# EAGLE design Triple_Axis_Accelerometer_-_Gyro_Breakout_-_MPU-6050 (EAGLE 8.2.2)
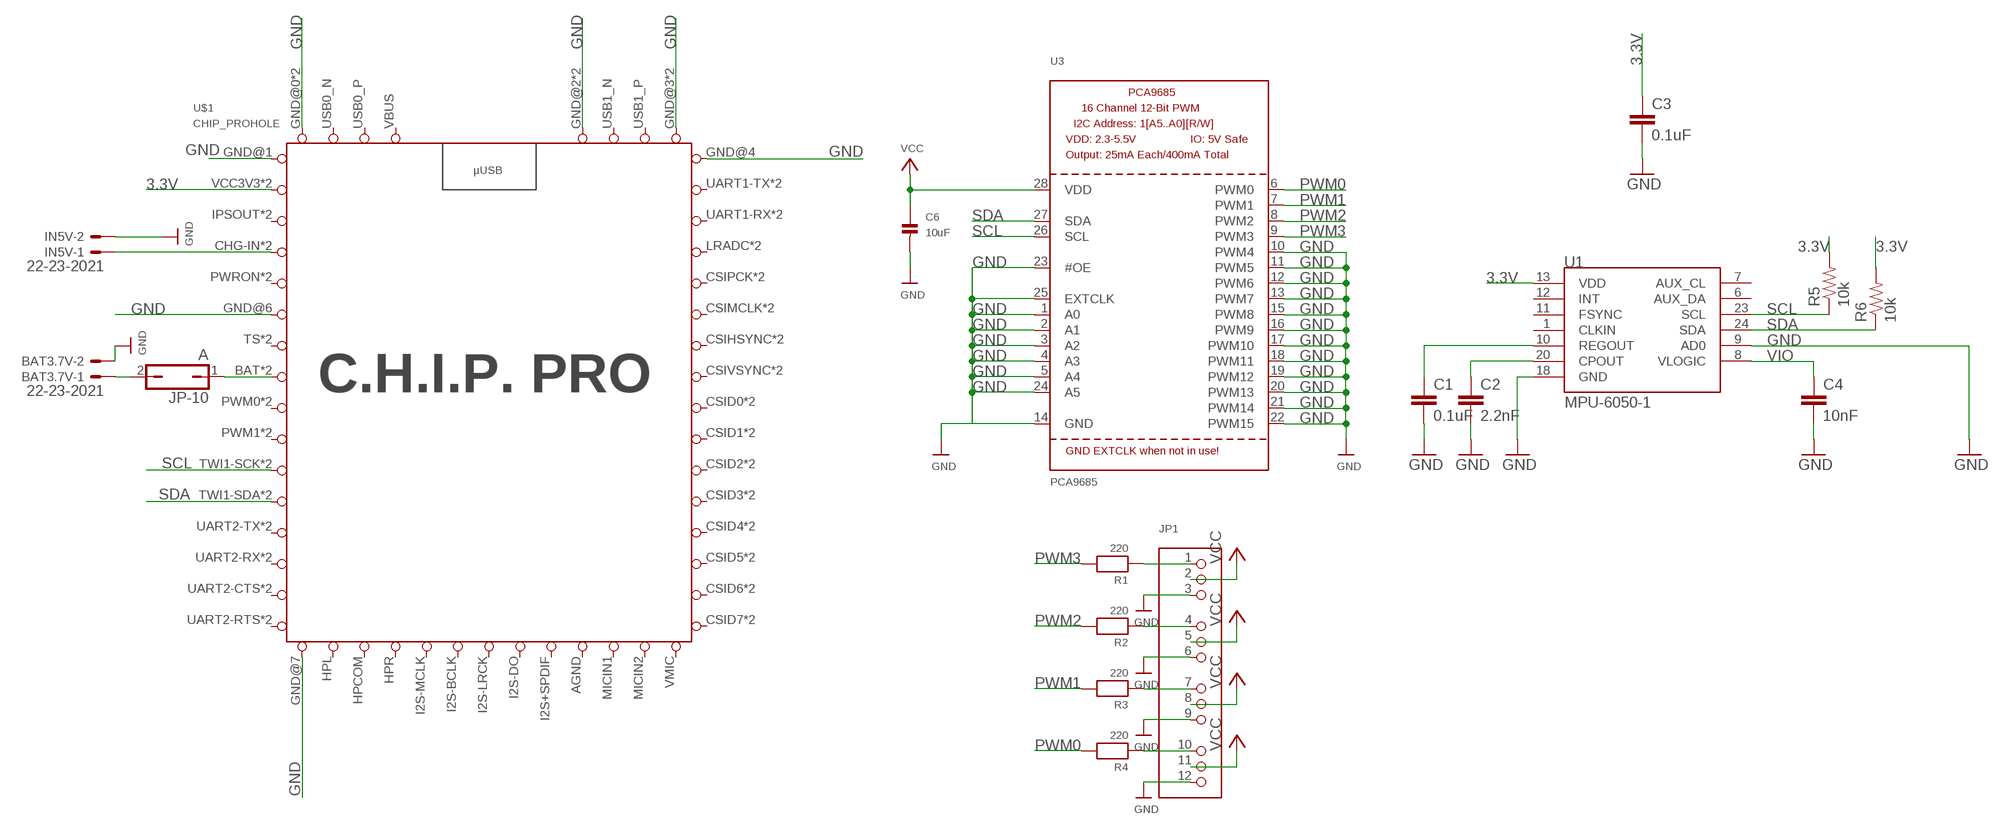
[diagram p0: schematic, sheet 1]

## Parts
BAT3.7V  22-23-2021  [22-23-2021]
C1  0.1uF  CAP0603-CAP  [0603-CAP]
C2  2.2nF  CAP0603-CAP  [0603-CAP]
C3  0.1uF  CAP0603-CAP  [0603-CAP]
C4  10nF  CAP0603-CAP  [0603-CAP]
C6  10uF  CAP_CERAMIC0805  [0805]
IN5V  22-23-2021  [22-23-2021]
JP1  HEADER-3X04  [3X04]
JP-10  A  JP1Q  [JP1]
R1  220  RESISTOR0805  [0805]
R2  220  RESISTOR0805  [0805]
R3  220  RESISTOR0805  [0805]
R4  220  RESISTOR0805  [0805]
R5  10k  R-US_R0805  [R0805]
R6  10k  R-US_R0805  [R0805]
U1  MPU-6050-1  [QFN-24-4MM2]
U3  PCA9685  [TSSOP28]
U$1  CHIP_PROHOLE  [CHIP_PRO_HOLE]

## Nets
3.3V: C3.1 R5.2 R6.2 U1.13(VDD) U$1.VCC3V3 U$1.VCC3V3-1(VCC3V3)
GND: BAT3.7V.2 C1.2 C2.2 C3.2 C4.2 C6.2 IN5V.2 JP1.3 JP1.6 JP1.9 JP1.12 U1.9(AD0) U1.18(GND) U3.1(A0) U3.2(A1) U3.3(A2) U3.4(A3) U3.5(A4) U3.10(PWM4) U3.11(PWM5) U3.12(PWM6) U3.13(PWM7) U3.14(GND) U3.15(PWM8) U3.16(PWM9) U3.17(PWM10) U3.18(PWM11) U3.19(PWM12) U3.20(PWM13) U3.21(PWM14) U3.22(PWM15) U3.23(#OE) U3.24(A5) U3.25(EXTCLK) U$1.GND@0(GND) U$1.GND@0-1(GND) U$1.GND@1(GND) U$1.GND@2(GND) U$1.GND@2-1(GND) U$1.GND@3(GND) U$1.GND@3-1(GND) U$1.GND@4(GND) U$1.GND@6(GND) U$1.GND@7(GND)
N$1: JP1.1 R1.1
N$2: JP1.4 R2.1
N$3: C2.1 U1.20(CPOUT)
N$4: JP1.7 R3.1
N$5: C1.1 U1.10(REGOUT)
N$6: JP1.10 R4.1
N$9: IN5V.1 U$1.CHG-IN U$1.CHG-IN-1(CHG-IN)
PWM0: R4.2 U3.6(PWM0)
PWM1: R3.2 U3.7(PWM1)
PWM2: R2.2 U3.8(PWM2)
PWM3: R1.2 U3.9(PWM3)
SCL: R5.1 U1.23(SCL) U3.26(SCL) U$1.TWI1-SCK U$1.TWI1-SCK-1(TWI1-SCK)
SDA: R6.1 U1.24(SDA) U3.27(SDA) U$1.TWI1-SDA U$1.TWI1-SDA-1(TWI1-SDA)
VCC: BAT3.7V.1 C6.1 JP1.2 JP1.5 JP1.8 JP1.11 JP-10.1 JP-10.2 U3.28(VDD) U$1.BAT U$1.BAT-1(BAT)
VIO: C4.1 U1.8(VLOGIC)
Unconnected: U1.1(CLKIN) U1.6(AUX_DA) U1.7(AUX_CL) U1.11(FSYNC) U1.12(INT) U$1.CSID0 U$1.CSID0-1(CSID0) U$1.CSID1 U$1.CSID1-1(CSID1) U$1.CSID2 U$1.CSID2-1(CSID2) U$1.CSID3 U$1.CSID3-1(CSID3) U$1.CSID4 U$1.CSID4-1(CSID4) U$1.CSID5 U$1.CSID5-1(CSID5) U$1.CSID6 U$1.CSID6-1(CSID6) U$1.CSID7 U$1.CSID7-1(CSID7) U$1.CSIHSYNC U$1.CSIHSYNC-1(CSIHSYNC) U$1.CSIMCLK U$1.CSIMCLK-1(CSIMCLK) U$1.CSIPCK U$1.CSIPCK-1(CSIPCK) U$1.CSIVSYNC U$1.CSIVSYNC-1(CSIVSYNC) U$1.HPCOM U$1.HPL U$1.HPR U$1.I2S+SPDIF(I2SSPDIF) U$1.I2S-BCLK(I2SBCLK) U$1.I2S-DO(I2SDO) U$1.I2S-LRCK(I2SLRCK) U$1.I2S-MCLK(I2SMCLK) U$1.LRADC U$1.LRADC-1(LRADC) U$1.MICIN1 U$1.MICIN2 U$1.PWM0 U$1.PWM0-1(PWM0) U$1.PWM1 U$1.PWM1-1(PWM1) U$1.PWRON U$1.PWRON-1(PWRON) U$1.TS U$1.TS-1(TS) U$1.UART1-RX U$1.UART1-RX-1(UART1-RX) U$1.UART1-TX U$1.UART1-TX-1(UART1-TX) U$1.UART2-CTS U$1.UART2-CTS-1(UART2-CTS) U$1.UART2-RTS U$1.UART2-RTS-1(UART2-RTS) U$1.UART2-RX U$1.UART2-RX-1(UART2-RX) U$1.UART2-TX U$1.UART2-TX-1(UART2-TX) U$1.USB0_N U$1.USB0_P U$1.USB1_N U$1.USB1_P U$1.VMIC

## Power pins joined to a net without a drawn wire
AGND: U$1.AGND
IPSOUT: U$1.IPSOUT U$1.IPSOUT-1(IPSOUT)
VBUS: U$1.VBUS

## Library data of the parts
BAT3.7V IN5V = con-molex:22-23-2021: .100" (2.54mm) Center Header - 2 Pin; MF: MOLEX; MPN: 22-23-2021; OC_FARNELL: 1462926; OC_NEWARK: 25C3832
C1-C4 = SparkFun:CAP: Capacitor
C6 = microbuilder:CAP_CERAMIC: Ceramic Capacitors
JP1 = microbuilder:HEADER-3X04
JP-10 = jumper:JP1Q: JUMPER
R1-R4 = microbuilder:RESISTOR: Resistors
R5 R6 = rcl:R-US_: RESISTOR, American symbol
U1 = Testing:MPU-6050
U3 = microbuilder:PCA9685: PCA9685 - 16 Channel 12-Bit I2C PWM Controller 5.0V tolerant 16 channel, 12-bit I2C PWM controller with 25mA per output (max. 400mA total) Digikey: 568-5931-1-ND
U$1 = CHIP_Pro-Footprint:CHIP_PRO

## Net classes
0 Default: width 0.203 mm
1 vcc: width 0.254 mm
2 GND: width 0.813 mm

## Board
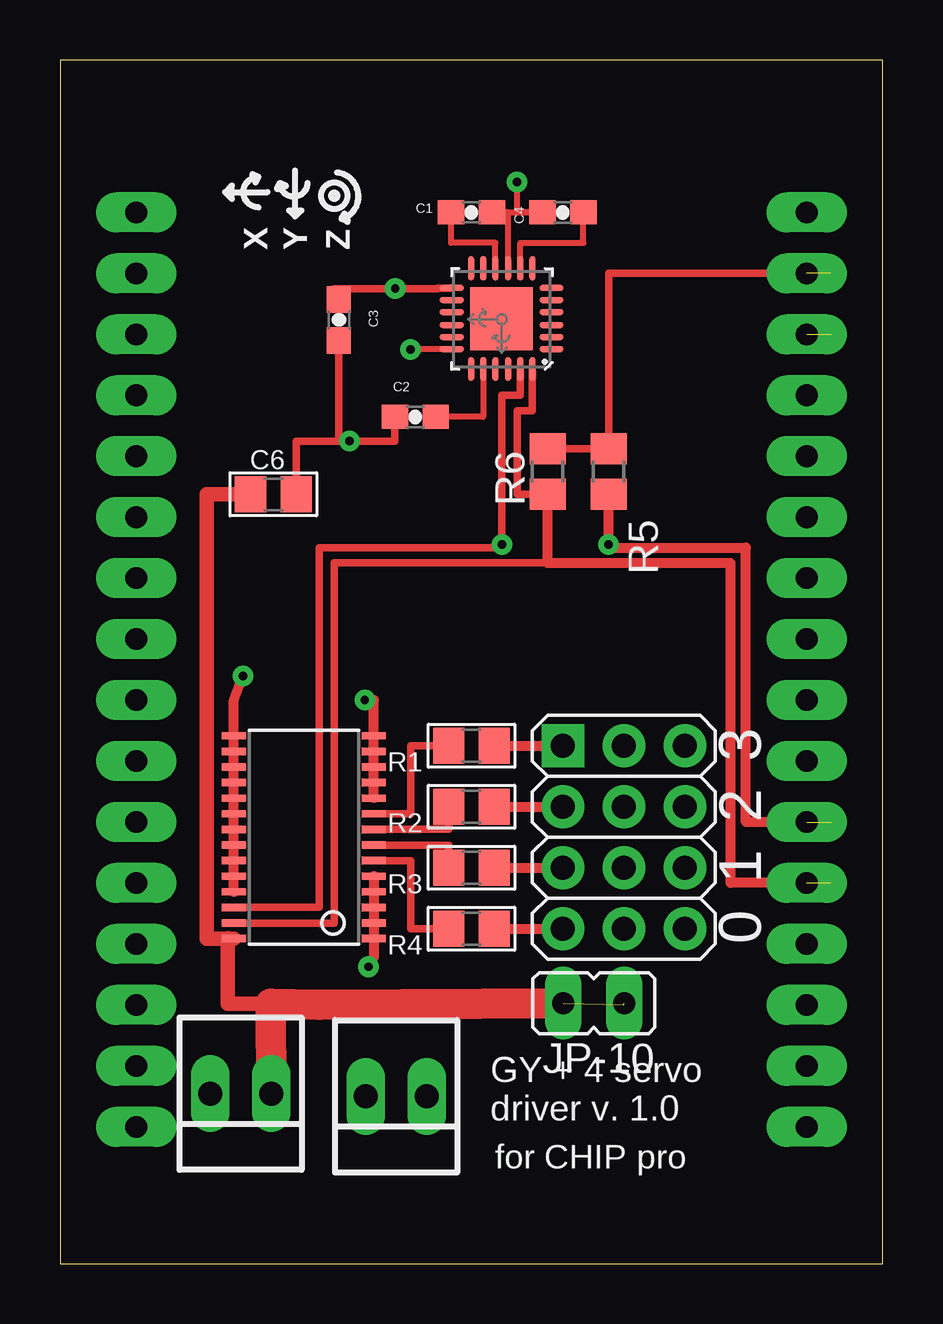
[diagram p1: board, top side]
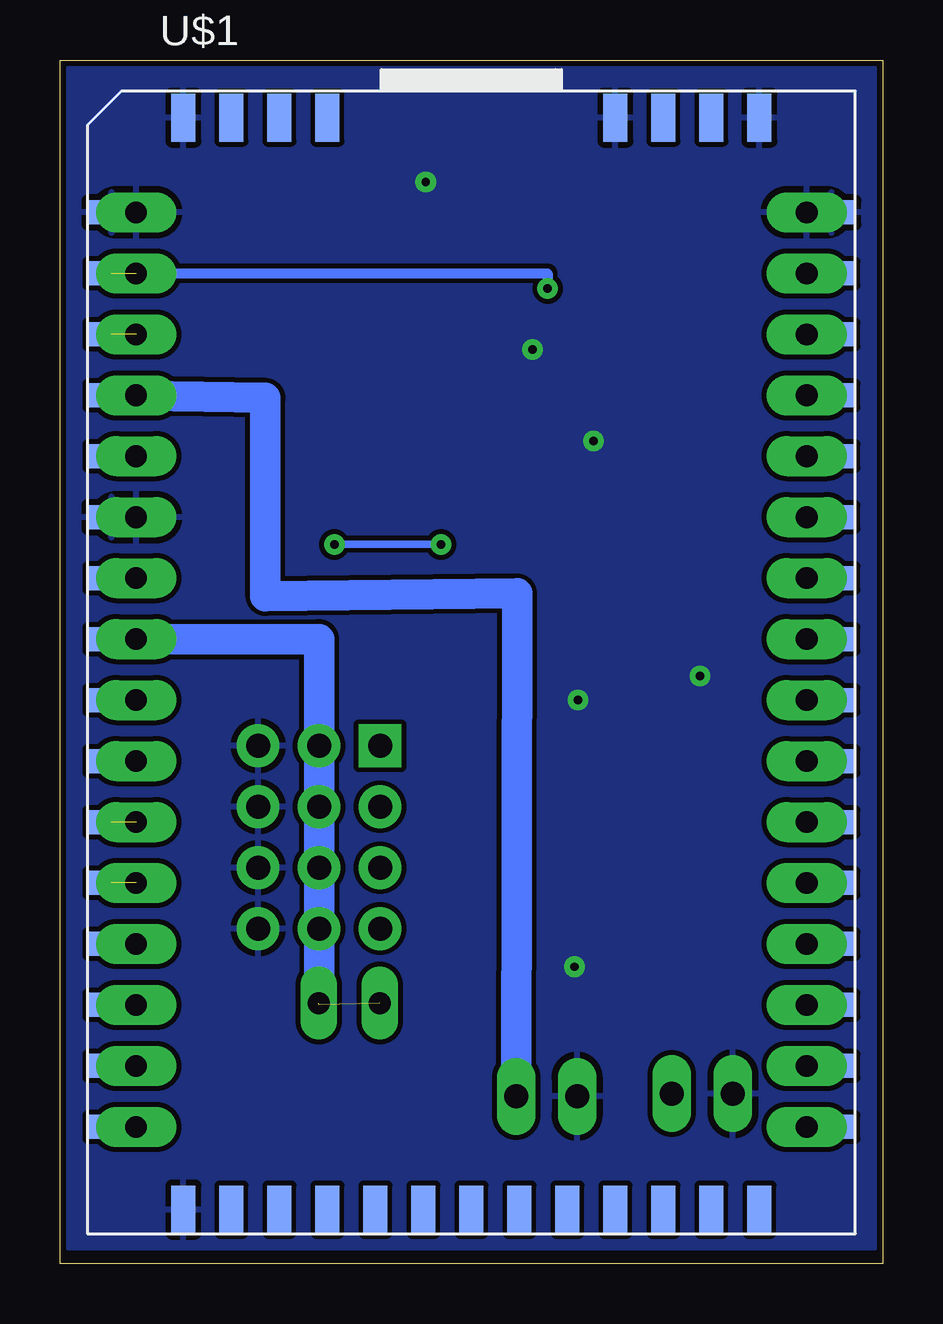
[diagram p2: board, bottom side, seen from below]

Size 34.29 x 50.17 mm. Coordinates in mm from the lower left corner, seen from the top.
Copper layers (1*16): Top 0.035mm / dielectric 1.5mm / Bottom 0.035mm
Design rules "SparkFun *": minimum track width 7mil, minimum drill 15mil, track to track 8mil, track to pad 8mil, pad to pad 8mil, via to via 8mil, smd to smd 8mil, copper to edge 8mil, drill to drill 8mil, minimum pad ring 12mil, minimum via ring 10mil, stop-mask expansion 4mil, vias tented up to drill 20mil, thermal gap 10mil
Milling: area 0,0 to 34.3,50.2

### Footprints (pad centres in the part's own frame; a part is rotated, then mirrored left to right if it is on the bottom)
22-23-2021 = drill 1 long: 1 -1.27,0; 2 1.27,0
0603-CAP = smd 1.1 x 1: 1 -0.85,0; 2 0.85,0
0805 = smd 1.3 x 1.5: 1 -0.95,0; 2 0.95,0
3X04 = drill 1 pad 1.778 square: 1 -3.81,-2.54 | drill 1 pad 1.778: 2 -3.81,0; 3 -3.81,2.54; 4 -1.27,-2.54; 5 -1.27,0; 6 -1.27,2.54; 7 1.27,-2.54; 8 1.27,0; 9 1.27,2.54; 10 3.81,-2.54; 11 3.81,0; 12 3.81,2.54
JP1 = drill 0.914 long: 1 0,-1.27; 2 0,1.27
R0805 = smd 1.3 x 1.5: 1 -0.95,0; 2 0.95,0
QFN-24-4MM2 = smd 1.016 x 0.254: 1 -2.066,1.257; 2 -2.066,0.75; 3 -2.066,0.247; 4 -2.066,-0.287; 5 -2.066,-0.792; 6 -2.066,-1.297; 13 2.086,-1.297; 14 2.086,-0.792; 15 2.086,-0.287; 16 2.086,0.247; 17 2.086,0.75; 18 2.086,1.257 | smd 0.254 x 1.016: 7 -1.267,-2.122; 8 -0.762,-2.122; 9 -0.258,-2.122; 10 0.278,-2.122; 11 0.78,-2.122; 12 1.287,-2.122; 19 1.287,2.082; 20 0.78,2.082; 21 0.278,2.082; 22 -0.258,2.082; 23 -0.762,2.082; 24 -1.267,2.082 | smd 2.616 x 2.616: P$1 0.02,-0.01
TSSOP28 = smd 0.305 x 0.991: 1 -4.225,-2.918; 2 -3.575,-2.918; 3 -2.925,-2.918; 4 -2.275,-2.918; 5 -1.625,-2.918; 6 -0.975,-2.918; 7 -0.325,-2.918; 8 0.325,-2.918; 9 0.975,-2.918; 10 1.625,-2.918; 11 2.275,-2.918; 12 2.925,-2.918; 13 3.575,-2.918; 14 4.225,-2.918; 15 4.225,2.918; 16 3.575,2.918; 17 2.925,2.918; 18 2.275,2.918; 19 1.625,2.918; 20 0.975,2.918; 21 0.325,2.918; 22 -0.325,2.918; 23 -0.975,2.918; 24 -1.625,2.918; 25 -2.275,2.918; 26 -2.925,2.918; 27 -3.575,2.918; 28 -4.225,2.918
CHIP_PRO_HOLE = smd 1 x 2: AGND 6,-22.5; GND@1 -12,-22.5; GND@4 -12,23; GND@6 6,23; GND@7 12,23; HPCOM -8,-22.5; HPL -10,-22.5; HPR -6,-22.5; I2S+SPDIF 4,-22.5; I2S-BCLK -2,-22.5; I2S-DO 2,-22.5; I2S-LRCK 0,-22.5; I2S-MCLK -4,-22.5; MICIN1 8,-22.5; MICIN2 10,-22.5; USB0_N -10,23; USB0_P -8,23; USB1_N 8,23; USB1_P 10,23; VBUS -6,23; VMIC 12,-22.5 | smd 2 x 1: BAT -15,1.27; CHG-IN -15,11.43; CSID0 15,-1.27; CSID1 15,-3.81; CSID2 15,-6.35; CSID3 15,-8.89; CSID4 15,-11.43; CSID5 15,-13.97; CSID6 15,-16.51; CSID7 15,-19.05; CSIHSYNC 15,3.81; CSIMCLK 15,6.35; CSIPCK 15,8.89; CSIVSYNC 15,1.27; GND@0 15,19.05; GND@2 -15,6.35; GND@3 -15,19.05; IPSOUT -15,13.97; LRADC 15,11.43; PWM0 -15,-1.27; PWM1 -15,-3.81; PWRON -15,8.89; TS -15,3.81; TWI1-SCK -15,-6.35; TWI1-SDA -15,-8.89; UART1-RX 15,13.97; UART1-TX 15,16.51; UART2-CTS -15,-16.51; UART2-RTS -15,-19.05; UART2-RX -15,-13.97; UART2-TX -15,-11.43; VCC3V3 -15,16.51 | drill 0.9 pad 1.676 long: BAT-1 -13.97,1.27; CHG-IN-1 -13.97,11.43; CSID0-1 13.97,-1.27; CSID1-1 13.97,-3.81; CSID2-1 13.97,-6.35; CSID3-1 13.97,-8.89; CSID4-1 13.97,-11.43; CSID5-1 13.97,-13.97; CSID6-1 13.97,-16.51; CSID7-1 13.97,-19.05; CSIHSYNC-1 13.97,3.81; CSIMCLK-1 13.97,6.35; CSIPCK-1 13.97,8.89; CSIVSYNC-1 13.97,1.27; GND@0-1 13.97,19.05; GND@2-1 -13.97,6.35; GND@3-1 -13.97,19.05; IPSOUT-1 -13.97,13.97; LRADC-1 13.97,11.43; PWM0-1 -13.97,-1.27; PWM1-1 -13.97,-3.81; PWRON-1 -13.97,8.89; TS-1 -13.97,3.81; TWI1-SCK-1 -13.97,-6.35; TWI1-SDA-1 -13.97,-8.89; UART1-RX-1 13.97,13.97; UART1-TX-1 13.97,16.51; UART2-CTS-1 -13.97,-16.51; UART2-RTS-1 -13.97,-19.05; UART2-RX-1 -13.97,-13.97; UART2-TX-1 -13.97,-11.43; VCC3V3-1 -13.97,16.51

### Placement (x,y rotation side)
BAT3.7V  7.52,7.1 180 top
C1  17.14,43.82 0 top
C2  14.81,35.29 180 top
C3  11.62,39.33 270 top
C4  20.95,43.82 180 top
C6  8.89,32.07 0 top
IN5V  14.01,6.99 180 top
JP1  23.49,17.78 270 top
JP-10  22.25,10.87 90 top
R1  17.14,21.59 180 top
R2  17.14,19.05 180 top
R3  17.14,16.51 180 top
R4  17.14,13.97 180 top
R5  22.86,33.02 90 top
R6  20.32,33.02 90 top
U1  18.41,39.37 180 top
U3  10.16,17.78 90 top
U$1  17.14,24.77 0 bottom

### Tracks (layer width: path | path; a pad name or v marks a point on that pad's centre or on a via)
3.3V  (via drill 0.35)  (1 unrouted)
  Top 0.305: U1.13 16.31,40.65 15.75,40.65 15.74,40.64 v13.97,40.64 11.43,40.64 11.43,40.18 C3.1 | R6.2 R5.2 22.86,41.28 U$1.VCC3V3-1
  Bottom 0.406: v13.97,40.64 13.97,41.28 U$1.VCC3V3
GND  (via drill 0.35)
  Top 0.254: U1.18 14.6,38.11 | U1.9 18.67,43.82 C1.2 C4.2 19.05,43.82 v19.05,45.09
  Top 0.305: C3.2 11.62,34.29 v12.06,34.29 | C6.2 9.84,34.29 v12.06,34.29 | C2.2 13.96,34.29 v12.06,34.29 | 14.6,38.11 v14.6,38.1
  Top 0.406: U3.25 U3.24 U3.23 U3.22 U3.21 U3.20 U3.19 U3.18 U3.17 U3.16 U3.15 7.24,23.5 v7.62,24.5 | U3.10 U3.11 U3.12 U3.13 U3.14 13.08,23.5 v12.7,23.5 | U3.5 U3.4 U3.3 U3.2 U3.1 13.08,12.8 v12.86,12.38
  pour Bottom: 33.97,49.85 33.97,0.64 0.32,0.64 0.32,49.85
IPSOUT  (1 unrouted)
N$1
  Top 0.406: R1.1 JP1.1
N$2
  Top 0.406: R2.1 JP1.4
N$3
  Top 0.254: U1.20 17.63,35.29 C2.1
N$4
  Top 0.406: R3.1 JP1.7
N$5
  Top 0.254: U1.10 18.14,42.55 16.29,42.55 C1.1
N$6
  Top 0.406: R4.1 JP1.10
N$9
  Bottom 1.27: IN5V.1 15.24,27.94 25.73,27.83 25.73,36.09 U$1.CHG-IN
PWM0
  Top 0.305: U3.6 14.6,16.81 14.6,13.97 R4.2
PWM1
  Top 0.305: U3.7 16.19,17.46 R3.2
PWM2
  Top 0.305: U3.8 16.19,18.11 R2.2
PWM3
  Top 0.305: U3.9 14.6,18.76 14.6,21.59 R1.2
SCL  (via drill 0.35)  (1 unrouted)
  Top 0.305: U3.26 10.79,14.86 10.79,29.85 18.41,29.85 v18.41,29.98 18.41,36.2 19.18,36.2 U1.23
  Top 0.406: U$1.TWI1-SCK-1 28.57,18.42 28.57,29.85 22.86,29.85 v22.86,29.98 R5.1
  Bottom 0.305: v18.41,29.98 v22.86,29.98
SDA  (1 unrouted)
  Top 0.305: U3.27 11.43,14.21 11.43,29.21 20.32,29.21 | R6.1 19.05,32.07 19.05,35.56 19.68,35.56 U1.24
  Top 0.406: R6.1 20.32,29.21 27.94,29.21 27.94,15.88 U$1.TWI1-SDA-1
VCC  (2 unrouted)
  Top 0.406: U3.28 6.98,13.56 6.98,12.97
  Top 0.61: 6.98,13.57 6.98,12.97 6.98,10.84 8.78,10.85 | U3.28 6.11,13.56 6.11,32.07 C6.1
  Top 1.27: BAT3.7V.1 8.78,10.85 10.79,10.81 JP-10.2
  Bottom 1.27: U$1.BAT 23.49,26.04 JP1.2 JP1.5 JP1.8 JP1.11 23.49,10.8
VIO
  Top 0.254: U1.8 19.18,42.55 21.8,42.55 C4.1

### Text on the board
tPlace: X | Y | Z | 3 | 2 | 1 | 0 | GY + 4 servo / driver v. 1.0 | for CHIP pro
